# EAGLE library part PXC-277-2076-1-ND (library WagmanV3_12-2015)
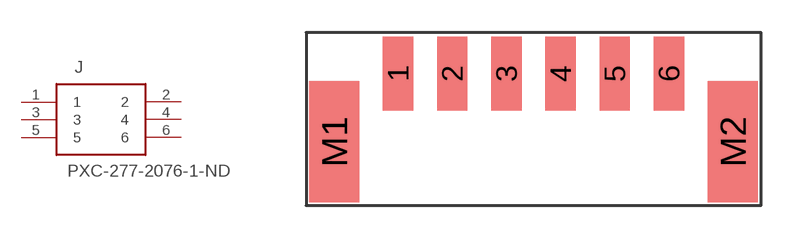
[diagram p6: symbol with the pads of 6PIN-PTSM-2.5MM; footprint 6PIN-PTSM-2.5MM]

Designator prefix J

## PXC-277-2076-1-ND  [6PIN-PTSM-2.5MM]
1  1
2  2
3  3
4  4
5  5
6  6

## Footprint 6PIN-PTSM-2.5MM (pad centres in mm)
smd 1.4 x 3.4: 1 -6.25,0; 2 -3.75,0; 3 -1.25,0; 4 1.25,0; 5 3.75,0; 6 6.25,0
smd 2.3 x 5.6: M1 -9.2,-3.15; M2 9.2,-3.15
